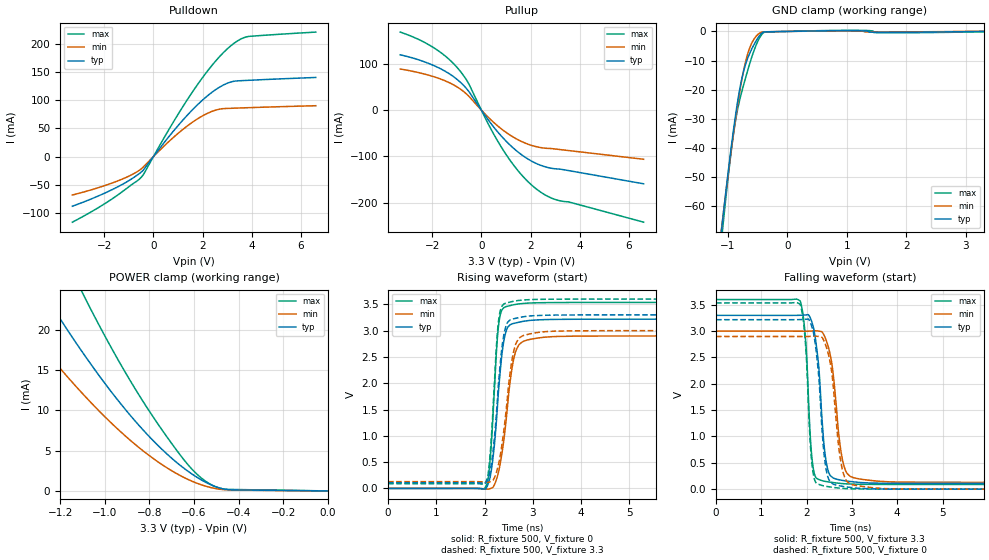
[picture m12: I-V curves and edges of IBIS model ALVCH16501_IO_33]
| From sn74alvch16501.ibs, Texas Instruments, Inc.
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[Model]   ALVCH16501_IO_33
Model_type  I/O
Vinl=0.8
Vinh=2.0
Enable   Active-Low
Vref =   0
Rref =   500
Cref =   50p
Vmeas =   1.5
| variable   typ   min   max
C_comp   3.01pF   2.45pF   3.36pF
| C_pullup   4.12pF   3.10pF   5.00pF
| C_pulldown   3.33pF   2.33pF   4.27pF
| C_tri-state   3.01pF   2.45pF   3.36pF
[Temperature Range]   40   100   -40
| Ambient temperature   25   85   -40
[Voltage range]   3.3   3   3.6
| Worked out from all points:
|   slope of the pulldown table from 0 to 0.495 V, typ, clamps not added: 17.6 ohm
|   slope of the pullup table from 0 to 0.495 V, typ, clamps not added: 13.7 ohm
|   GND clamp passes 1 mA (typ) near -0.45 V on its own axis
|   POWER clamp passes 1 mA (typ) near -0.54 V on its own axis
|   rising waveform, R_fixture 500, V_fixture 0: 20-80 % time 181ps typ, 230ps min, 135ps max; typ from 0 V to 3.22 V
|   falling waveform, R_fixture 500, V_fixture 3.3: 20-80 % time 172ps typ, 213ps min, 126ps max; typ from 3.3 V to 0.109 V
|   rising waveform, R_fixture 500, V_fixture 3.3: 20-80 % time 178ps typ, 227ps min, 133ps max; typ from 0.109 V to 3.3 V
|   falling waveform, R_fixture 500, V_fixture 0: 20-80 % time 171ps typ, 207ps min, 125ps max; typ from 3.22 V to 0 V
[GND Clamp]
| ALVCH16501_IO_33
|   Voltage   I(typ)   I(min)   I(max)
-3.3V     -525.1mA   -495.7mA   -572.2mA
-1.11V    -68.65mA   -68.11mA   -72.05mA
-1.09V    -64.99mA   -64.68mA   -68.03mA
-1.07V    -61.37mA   -61.28mA   -64.08mA
-970mV    -44.01mA   -44.85mA   -45.45mA
-890mV    -31.43mA   -32.66mA   -33.03mA
-770mV    -16.63mA   -17.04mA   -20.93mA
-700mV    -11.11mA   -10.21mA   -15.72mA
-620mV    -6.918mA   -4.99mA    -10.18mA
-445mV    -889.9uA   -352.3uA   -1.449mA
775mV     221.7uA    143.3uA    341.2uA
3.3V      943.9pA    66.99uA    -116.8uA
[POWER Clamp]
| ALVCH16501_IO_33
|   Voltage   I(typ)   I(min)   I(max)
-3.3V     141.2mA    107.5mA    192.6mA
-1.475V   33.97mA    24.8mA     47.49mA
-1.45V    32.75mA    23.87mA    45.84mA
-1.265V   24.17mA    17.34mA    34.13mA
-1.105V   17.4mA     12.23mA    24.83mA
-1.085V   16.6mA     11.63mA    23.73mA
-945mV    11.38mA    7.748mA    16.48mA
-810mV    7.013mA    4.577mA    10.3mA
-660mV    3.13mA     1.88mA     4.383mA
-565mV    1.329mA    738.8uA    1.547mA
-460mV    200.7uA    146.2uA    210.2uA
-48.03fV  943.9pA    48.42nA    50.47pA
[Pulldown]
| ALVCH16501_IO_33
|   Voltage   I(typ)   I(min)   I(max)
-3.3V     -88.13mA   -68.24mA   -116.5mA
-1.53V    -55.44mA   -44.53mA   -70.64mA
-910mV    -40.25mA   -32.85mA   -50.64mA
-495mV    -27.48mA   -21.72mA   -36.66mA
745mV     41.65mA    31.4mA     56.6mA
1.69V     87.56mA    64.04mA    121.3mA
2.485V    117.4mA    81.78mA    167.3mA
2.87V     127.5mA    85.16mA    185.5mA
3.215V    133.1mA    85.74mA    198.9mA
3.56V     134.6mA    86.29mA    208.7mA
3.865V    135.3mA    86.74mA    213.1mA
6.6V      140.4mA    90.22mA    220.9mA
[Pullup]
| ALVCH16501_IO_33
|   Voltage   I(typ)   I(min)   I(max)
-3.3V     119.7mA    88.95mA    168.8mA
-2.535V   108.5mA    80.93mA    152.5mA
-1.96V    97mA       72.73mA    135.7mA
-1.42V    82.48mA    62.16mA    114.8mA
-970mV    65.69mA    49.61mA    91.25mA
-540mV    42.39mA    31.64mA    59.51mA
315mV     -23.69mA   -17.32mA   -33.48mA
945mV     -63.75mA   -45.87mA   -91.13mA
1.59V     -94.67mA   -66.7mA    -137.3mA
2.235V    -115.4mA   -79.06mA   -170.5mA
3.04V     -127.1mA   -84.3mA    -193.9mA
6.6V      -159.3mA   -106.3mA   -242.4mA
[Ramp]
| ALVCH16501_IO_33
| variable   typ   min   max
dV/dt_r   1.94/1.91E-10   1.75/2.41E-10   2.13/1.39E-10
dV/dt_f   1.92/1.84E-10   1.73/2.14E-10   2.11/1.30E-10
R_load = 500
[Rising Waveform]
| ALVCH16501_IO_33
R_fixture =   500
C_fixture =   0
L_fixture =   0
V_fixture =   0
V_fixture_min = 0
V_fixture_max = 0
|   Time   V(typ)   V(min)   V(max)
0s        103.5pV    2.715nV    81.35pV
2ns       -11.17mV   -6.994mV   -194.5uV
2.06ns    52.47mV    -13.65mV   105.2mV
2.11ns    192.6mV    -6.193mV   493.1mV
2.255ns   1.399V     195.7mV    2.721V
2.32ns    2.18V      448.5mV    3.279V
2.44ns    2.969V     1.239V     3.455V
2.6ns     3.136V     2.442V     3.491V
2.85ns    3.183V     2.811V     3.52V
50ns      3.218V     2.899V     3.536V
[Falling Waveform]
| ALVCH16501_IO_33
R_fixture =   500
C_fixture =   0
L_fixture =   0
V_fixture =   3.3
V_fixture_min = 3
V_fixture_max = 3.6
|   Time   V(typ)   V(min)   V(max)
0s        3.3V       3V         3.6V
1.86ns    3.302V     2.999V     3.572V
1.97ns    3.308V     2.999V     2.915V
2.045ns   3.308V     2.999V     1.633V
2.17ns    2.986V     3.007V     297.6mV
2.45ns    435.6mV    2.782V     142.2mV
2.565ns   227.7mV    2.335V     127.7mV
2.79ns    166.8mV    563.2mV    105.9mV
4.175ns   110.1mV    132.6mV    89.17mV
50ns      109.1mV    128.8mV    89.01mV
[Rising Waveform]
| ALVCH16501_IO_33
R_fixture =   500
C_fixture =   0
L_fixture =   0
V_fixture =   3.3
V_fixture_min = 3
V_fixture_max = 3.6
|   Time   V(typ)   V(min)   V(max)
0s        109.1mV    128.8mV    89.01mV
2ns       98.54mV    121.5mV    89.44mV
2.105ns   288.7mV    122.3mV    536.3mV
2.18ns    748.3mV    159.4mV    1.592V
2.25ns    1.476V     317.6mV    2.758V
2.32ns    2.32V      598.1mV    3.357V
2.435ns   3.058V     1.38V      3.521V
2.59ns    3.223V     2.547V     3.556V
2.835ns   3.268V     2.915V     3.584V
50ns      3.3V       3V         3.6V
[Falling Waveform]
| ALVCH16501_IO_33
R_fixture =   500
C_fixture =   0
L_fixture =   0
V_fixture =   0
V_fixture_min = 0
V_fixture_max = 0
|   Time   V(typ)   V(min)   V(max)
0s        3.218V     2.899V     3.536V
1.86ns    3.22V      2.898V     3.506V
1.965ns   3.224V     2.898V     2.871V
2.04ns    3.23V      2.899V     1.59V
2.16ns    2.933V     2.905V     231mV
2.44ns    335mV      2.684V     52.46mV
2.555ns   116.3mV    2.224V     37.68mV
2.765ns   57.74mV    474.6mV    16.51mV
4.07ns    1.097mV    3.971mV    229.4uV
50ns      -868.4pV   2.133nV    -825.8pV
